(* Logix 5000 AddOnInstructionDefinition export; software revision 16.04 *)

TYPE ST_IOL_Error :   // IO-Link error codes
STRUCT
   nCommunicationError : DINT;   // Communication error
   nBlockError : INT;   // Function block error
   nIOLMError : INT;   // IO-Link master error
   nIOLError : INT;   // IO-Link device error
   iISDUIndex : DINT;   // IO-Link ISDU number
END_STRUCT
END_TYPE

TYPE STRING16 :   // string type
STRUCT
   LEN : DINT;
   DATA : SINT[16];
END_STRUCT
END_TYPE

TYPE STRING64 :   // string type
STRUCT
   LEN : DINT;
   DATA : SINT[64];
END_STRUCT
END_TYPE

TYPE STRING5 :   // string type
STRUCT
   LEN : DINT;
   DATA : SINT[5];
END_STRUCT
END_TYPE

TYPE ST_IOL_Data :   // Message elements and IO-Link record
STRUCT
   msgSource : SINT[255];   // Message: Source element
   msgDestination : SINT[255];   // Message: Destination element
   IOL_Record : SINT[232];   // IO-Link Record
END_STRUCT
END_TYPE

TYPE STRING8 :   // string type
STRUCT
   LEN : DINT;
   DATA : SINT[8];
END_STRUCT
END_TYPE

TYPE ST_PARKER_P8S :   // This data type includes the values of the IO-Link device
STRUCT
   VendorName : STRING16;   // ISDU 16: Vendor Name [String]
   ProductName : STRING16;   // ISDU 18: Product Name [String]
   VendorText : STRING64;   // ISDU 17: Vendor Text [String]
   ProductID : STRING64;   // ISDU 19: Product ID [String]
   ProductText : STRING64;   // ISDU 20: Product Text [String]
   SerialNumber : STRING8;   // ISDU 21: Serial Number [String]
   HWVersion : STRING5;   // ISDU 22: Hardware Version [String]
   FWVersion : STRING5;   // ISDU 23: Firmware Version [String]
   AppliName : STRING16;   // ISDU 24: Application Specific Tag [String]
   SysCommand : SINT;   // ISDU 2: Standard Command [Unsigned Integer]
   KeyLock : SINT;   // ISDU 81: Key Lock [Unsigned Integer]
END_STRUCT
END_TYPE

ADD_ON_INSTRUCTION FB_IOL_CALL_EIP   (* revision 3.1, vendor IO-Link *)
// This routine supports the communication between an IO-Link master and a Rockwell PLC via Ethernet/IP.
// Help:
// This routine supports the communication between an IO-Link master and a Rockwell PLC via Ethernet/IP. It makes it possible to read or write IO-Link variables (ISDUs) adressed via index and subindex.
// The function block supports the following EtherNet/IP IO-Link Masters:
// - SICK IOLG2EI (MasterType 0)
// - Balluff BNI EIP (MasterType 0)
// - Phoenix Axioline (MasterType 1)
// - Comtrol IOLM (MasterType 2)
// - Rockwell 1743-4IOL (MasterType 3)
VAR_IN_OUT
   msgCommunication_1 : MESSAGE; {required}   // Message instance for communication 1
   msgCommunication_2 : MESSAGE; {required}   // Message instance for communication 2
END_VAR
VAR_INPUT
   MasterType : SINT; {required}   // Type of the IO-Link master (0= SICK Master)
   PortNumber : SINT; {required}   // IO-Link port number (starting with 1)
   TimeOut : DINT; {visible}   // Time out time in [ms]
   Req : BOOL; {visible}   // Starts a request by a rising edge
   RW : BOOL; {visible}   // Read/Write selection (0= Read/ 1=Write)
   IOLIndex : DINT; {visible}   // IO-Link Index
   IOLSubIndex : INT; {visible}   // IO-Link Sub-Index
   Length : DINT; {visible}   // Byte-Length of the data that shold be written
END_VAR
VAR_OUTPUT
   ReadLength : DINT; {visible}   // Byte-Length of the read data
   Done : BOOL; {visible}   // Job done
   Busy : BOOL; {visible}   // Job busy
   Error : BOOL; {visible}   // Error detected (see Errorcode for more details)
END_VAR
VAR_IN_OUT
   Errorcode : ST_IOL_Error; {required}
   Data : ST_IOL_Data; {required}   // Data
END_VAR
VAR
   stTempError : ST_IOL_Error;
   iTemp1 : INT;   // Temporariliy variable
   iStep : INT;   // Current AOI step
   fbTriggerReq : FBD_ONESHOT;   // Instance: Edge detection (Req)
   fbTriggerMsgError2 : FBD_ONESHOT;   // Instance: Edge detection (MsgError2)
   fbTriggerMsgError1 : FBD_ONESHOT;   // Instance: Edge detection (MsgError1)
   fbTimeOut : FBD_TIMER;   // Instance: Time out
END_VAR

ROUTINE Logic   (* structured text *)
   (*=================================================================================
   Name: FB_IOL_Call_EIP
   Author: IO-Link
   -----------------------------------------------------------------------------------
   Description:
   This AOI supports the communication between an IO-Link master and a Rockwell
   PLC via Ethernet/IP. It makes it possible to read or write IO-Link variables (ISDUs)
   addressed via index and subindex.
   
   The function block supports the following EtherNet/IP IO-Link Masters:
   - SICK IOLG2EI          (MasterType 0)
   - Balluff BNI EIP       (MasterType 0)
   - Phoenix Axioline      (MasterType 1)
   - Comtrol IOLM          (MasterType 2)
   - Rockwell 1743-4IOL    (MasterType 3)
   
   -----------------------------------------------------------------------------------
   Version history:
   Date        | Version | Author  | Remark
   -----------------------------------------------------------------------------------
   03/08/2015  | 1.0     | IO-Link | Release version
   12/10/2015  | 2.0     | IO-Link | Support Phoenix IOLM
   04/02/2016  | 2.1     | IO-Link | Support Comtrol IOLM
   01/04/2016  | 2.2     | IO-Link | Support RA 1734 4IOL
   30/11/2016  | 3.0     | IO-Link | Error code extension
   25/04/2017  | 3.1     | IO-Link | Fix blocking of the MSG boxes
   ==================================================================================*)
   
   
   (*========== General ==========*)
   (*Initialize*)
   IF s:Fs THEN
   	Done:= 0;
   	Busy:= 0;
   	Error:= 0;
   	Errorcode.nCommunicationError:= 0;
   	Errorcode.nBlockError:= 0;
   	Errorcode.nIOLMError:= 0;
   	Errorcode.nIOLError:= 0;
   	Errorcode.iISDUIndex:= 0;
   	iStep:= 0;
   END_IF;
   
   (*Rising edge detection*)
   fbTriggerReq.InputBit:= Req;
   fbTriggerMsgError1.InputBit:= msgCommunication_1.ER;
   fbTriggerMsgError2.InputBit:= msgCommunication_2.ER;
   OSRI(fbTriggerReq);
   OSRI(fbTriggerMsgError1);
   OSRI(fbTriggerMsgError2);
   
   (*Error detetion*)
   IF (stTempError.nCommunicationError <>0 OR stTempError.nBlockError <>0 OR stTempError.nIOLMError <>0 OR stTempError.nIOLError <>0) AND Busy THEN
   	Errorcode.nCommunicationError:= stTempError.nCommunicationError;
   	Errorcode.nBlockError:= stTempError.nBlockError;
   	Errorcode.nIOLMError:= stTempError.nIOLMError;
   	Errorcode.nIOLError:= stTempError.nIOLError;
   	Errorcode.iISDUIndex:= stTempError.iISDUIndex;
   	stTempError.nCommunicationError:= 0;
   	stTempError.nBlockError:= 0;
   	stTempError.nIOLMError:= 0;
   	stTempError.nIOLError:= 0;
   	stTempError.iISDUIndex:= 0;
   
   	Done:= 0;
   	Busy:= 0;
   	Error:= 1;
   	iStep:= 0;
   	TND();
   END_IF;
   
   (*Time out detection*)
   fbTimeOut.TimerEnable:= Busy;
   fbTimeOut.PRE:= TimeOut;
   TONR(fbTimeOut);
   IF fbTimeOut.DN THEN
   	stTempError.nBlockError:= 16#0900; (*Error: Timeout*)
   	stTempError.iISDUIndex:= IOLIndex;
   	TND();
   END_IF;
   
   (*Get explicit messaging errors*)
   IF fbTriggerMsgError1.OutputBit THEN
   	stTempError.nCommunicationError:= (msgCommunication_1.EXERR * 65536) XOR msgCommunication_1.ERR;
   	stTempError.iISDUIndex:= IOLIndex;
   	TND();
   END_IF;
   
   (*Get explicit messaging errors*)
   IF fbTriggerMsgError2.OutputBit THEN
   	stTempError.nCommunicationError:= (msgCommunication_2.EXERR * 65536) XOR msgCommunication_2.ERR;
   	stTempError.iISDUIndex:= IOLIndex;
   	TND();
   END_IF;
   
   (*========== Send a new request ==========*)
   IF fbTriggerReq.OutputBit AND NOT Busy THEN
   	Done:= 0;
   	Busy:= 1;
   	Error:= 0;
   	Errorcode.nCommunicationError:= 0;
   	Errorcode.nBlockError:= 0;
   	Errorcode.nIOLMError:= 0;
   	Errorcode.nIOLError:= 0;
   	Errorcode.iISDUIndex:= 0;
   
   	iStep:= 1; (*Next step*)
   	TND();
   END_IF;
   
   
   (*========== Check parameter values ==========*)
   IF iStep =1 THEN
   
   	(*Check time out time*)
   	IF TimeOut <= 0 THEN
   		stTempError.nBlockError:= 16#0800; (*Error: Invalid time out time*)
   		stTempError.iISDUIndex:= IOLIndex;
   		TND();
   
   	(*Check port number*)
   	ELSIF PortNumber < 1 THEN
   		stTempError.nBlockError:= 16#0400; (*Error: Port number < 1*)
   		stTempError.iISDUIndex:= IOLIndex;
   		TND();
   
   	(*Check index*)
   	ELSIF IOLIndex < 0 OR IOLIndex > 32767 THEN
   		stTempError.nBlockError:= 16#0100; (*Error: 0 > Index > 32767*)
   		stTempError.iISDUIndex:= IOLIndex;
   		TND();
   
   	(*Check sub-index*)
   	ELSIF IOLSubIndex < 0 OR IOLSubIndex >255 THEN
   		stTempError.nBlockError:= 16#0300; (*Error: 0 > Sub-Index > 255*)
   		stTempError.iISDUIndex:= IOLIndex;
   		TND();
   
   	(*Check length*)
   	ELSIF Length < 0 OR Length > 232 THEN
   		stTempError.nBlockError:= 16#0200; (*Error: 0 > Length > 232*)
   		stTempError.iISDUIndex:= IOLIndex;
   		TND();
   	END_IF;
   
   	(*Check master type*)
   	IF MasterType = 0 THEN (*SICK*)
   		iStep:= 10; (*Next step*)
   	ELSIF MasterType = 1 THEN (*Phoenix*)
   		iStep:= 20;
   	ELSIF MasterType = 2 THEN (*Comtrol*)
   		iStep:= 30;
   	ELSIF MasterType = 3 THEN (*RA*)
   		iStep:= 40;
   	ELSE
   		stTempError.nBlockError:= 16#0600; (*Error: Master type <> 0*)
   		TND();
   	END_IF;
   END_IF;
   
   
   (*********** SICK IO-Link Master***********)
   (*========== Send a request ==========*)
   IF iStep =10 AND NOT msgCommunication_1.EW AND NOT msgCommunication_1.ST THEN
   	(*Define message parameter*)
   	msgCommunication_1.Class:= 150; (*Fix 0x96*)
   	msgCommunication_1.Instance:= PortNumber; (*Port starts at 1*)
   
   	(*Define index and subindex*)
   	COP(IOLIndex, Data.msgSource[0], 2); (*Index*)
   	Data.msgSource[2]:= IOLSubIndex; (*Sub-Index*)
   
   	(*Add attribute and payload*)
   	IF RW THEN
   		msgCommunication_1.Attribute:= 2; (*Write ISDU*)
   		msgCommunication_1.REQ_LEN:= 3 + Length; (*Byte length of the request*)
   		COP(Data.IOL_Record[0], Data.msgSource[3],Length); (*Payload*)
   	ELSE
   		msgCommunication_1.Attribute:= 3; (*Read ISDU*)
   		msgCommunication_1.REQ_LEN:= 3; (*Byte length of the request*)
   	END_IF;
   
   	(*Send request*)
   	MSG(msgCommunication_1);
   	iStep:= 11; (*Next step*)
   	TND();
   END_IF;
   
   
   (*========== Wait for reponse ==========*)
   IF iStep =11 THEN
   	IF fbTriggerMsgError1.OutputBit THEN
   		stTempError.nCommunicationError:= (msgCommunication_1.EXERR * 65536) XOR msgCommunication_1.ERR;
   		TND();
   	ELSIF msgCommunication_1.DN THEN
   		(*Valid response*)
   		IF Data.msgDestination[0] = 0 THEN
   			(*Write response*)
   			IF msgCommunication_1.Attribute = 2 THEN
   				iStep:= 2; (*Next step*)
   
   			(*Read response*)
   			ELSIF msgCommunication_1.Attribute = 3 THEN
   				ReadLength:= msgCommunication_1.DN_LEN - 1; (*Length of the response data*)
   				COP(Data.msgDestination[1], Data.IOL_Record[0], ReadLength);
   				iStep:= 2; (*Next step*)
   			END_IF;
   
   		(*IO-Link error detected*)
   		ELSIF Data.msgDestination[0] = -128 THEN
   			COP(Data.msgDestination[1], iTemp1, 2); (*Error: IO-Link Master*)
   			SWPB(iTemp1, REVERSE,stTempError.nIOLMError);
   			COP(Data.msgDestination[3], iTemp1, 2); (*Error: IO-Link Device*)
   			SWPB(iTemp1, REVERSE,stTempError.nIOLError);
   			TND();
   
   		(*Invalid response*)
   		ELSE
   			stTempError.nBlockError:= 16#0500; (*Error: Unknown response*)
   			stTempError.iISDUIndex:= IOLIndex;
   			TND();
   		END_IF;
   	END_IF;
   END_iF;
   
   
   (*********** Phoenix IO-Link Master***********)
   (*========== Read/Write handling ==========*)
   IF iStep = 20 AND NOT msgCommunication_1.EW AND NOT msgCommunication_1.ST AND NOT msgCommunication_2.EW AND NOT msgCommunication_2.ST THEN
   	(*Define message parameter*)
   	msgCommunication_1.Class:= 128; (*Fix 0x80*)
   	msgCommunication_1.Instance:= 1; (*Fix*)
   	msgCommunication_1.Attribute:= PortNumber; (*Port starts at 1*)
   	msgCommunication_2.Class:= 128; (*Fix 0x80*)
   	msgCommunication_2.Instance:= 1; (*Fix*)
   	msgCommunication_2.Attribute:= PortNumber; (*Port starts at 1*)
   
   	(*Define index and subindex*)
   	COP(IOLIndex, Data.msgSource[0], 2); (*Index*)
   	Data.msgSource[2]:= IOLSubIndex; (*Sub-Index*)
   
   	IF RW THEN
   		iStep:= 23; (*Next step*)
   	ELSE
   		iStep:= 21; (*Next step*)
   	END_IF;
   END_IF;
   
   
   
   (*========== Read ISDU ==========*)
   IF iStep = 21 THEN
   	msgCommunication_1.REQ_LEN:= 3; (*Byte length of the request*)
   
   	(*Send request*)
   	MSG(msgCommunication_1);
   	iStep:= 22; (*Next step*)
   END_IF;
   
   
   (*========== Wait for read reponse ==========*)
   IF iStep = 22 THEN
   	IF fbTriggerMsgError1.OutputBit THEN
   		stTempError.nCommunicationError:= (msgCommunication_1.EXERR * 65536) XOR msgCommunication_1.ERR;
   		stTempError.iISDUIndex:= IOLIndex;
   		IF msgCommunication_1.ERR = 30 THEN
   			COP(Data.msgDestination[0], stTempError.nIOLMError, 2); (*Error: IO-Link Device*)
   			COP(Data.msgDestination[2], iTemp1, 2); (*Error: IO-Link Device*)
   			SWPB(iTemp1, REVERSE,stTempError.nIOLError);
   			TND();
   		END_IF;
   	ELSIF msgCommunication_1.DN THEN
   		ReadLength:= msgCommunication_1.DN_LEN; (*Length of the response data*)
   		COP(Data.msgDestination[0], Data.IOL_Record[0], ReadLength);
   		iStep:= 2; (*Next step*)
   	END_IF;
   END_IF;
   
   
   (*========== Write ISDU ==========*)
   IF iStep = 23 THEN
   	msgCommunication_2.REQ_LEN:= 3 + Length; (*Byte length of the request*)
   	COP(Data.IOL_Record[0], Data.msgSource[3],Length); (*Payload*)
   
   	(*Send request*)
   	MSG(msgCommunication_2);
   	iStep:= 24; (*Next step*)
   END_IF;
   
   
   (*========== Wait for write reponse ==========*)
   IF iStep = 24 THEN
   	IF fbTriggerMsgError2.OutputBit THEN
   		stTempError.nCommunicationError:= (msgCommunication_2.EXERR * 65536) XOR msgCommunication_2.ERR;
   		stTempError.iISDUIndex:= IOLIndex;
   		IF msgCommunication_2.ERR = 30 THEN
   			COP(Data.msgDestination[0], stTempError.nIOLMError, 2); (*Error: IO-Link Device*)
   			COP(Data.msgDestination[2], iTemp1, 2); (*Error: IO-Link Device*)
   			SWPB(iTemp1, REVERSE,stTempError.nIOLError);
   			TND();
   		END_IF;
   	ELSIF msgCommunication_2.DN THEN
   		iStep:= 2; (*Next step*)
   	END_IF;
   END_IF;
   
   
   (*********** Comtrol IO-Link Master***********)
   (*========== Send a request ==========*)
   IF iStep = 30 AND NOT msgCommunication_1.EW AND NOT msgCommunication_1.ST THEN
   	(*Define message parameter*)
   	msgCommunication_1.Class:= 116; (*Fix 0x74*)
   	msgCommunication_1.Instance:= PortNumber; (*Port starts at 1*)
   	msgCommunication_1.Attribute:= 1; (*Fix*)
   	Data.msgSource[0]:= 0; (*No byte swapping*)
   
   	(*Define index and subindex*)
   	COP(IOLIndex, Data.msgSource[2], 2); (*Index*)
   	Data.msgSource[4]:= IOLSubIndex; (*Sub-Index*)
   	Data.msgSource[5]:= 0; (*Sub-Index*)
   	msgCommunication_1.REQ_LEN:= 240; (*Byte length of the request = 232 + 8*)
   
   	(*Add attribute and payload*)
   	IF RW THEN
   		Data.msgSource[1]:= 2; (*Write operation*)
   		COP(Length, Data.msgSource[6], 2); (*Length*)
   		COP(Data.IOL_Record[0], Data.msgSource[8], Length); (*Payload*)
   	ELSE
   		Data.msgSource[1]:= 1; (*Read operation*)
   		Data.msgSource[6]:= -24; (*Max IO-Link length*)
   		Data.msgSource[7]:= 0;
   	END_IF;
   
   	(*Send request*)
   	MSG(msgCommunication_1);
   	iStep:= 31; (*Next step*)
   	TND();
   END_IF;
   
   
   (*========== Wait for reponse ==========*)
   IF iStep = 31 THEN
   	IF fbTriggerMsgError1.OutputBit THEN
   		stTempError.nCommunicationError:= (msgCommunication_1.EXERR * 65536) XOR msgCommunication_1.ERR;
   		stTempError.iISDUIndex:= IOLIndex;
   		TND();
   	ELSIF msgCommunication_1.DN THEN
   		(*Valid response*)
   		IF Data.msgDestination[0] = 32 THEN
   			(*Write response*)
   			IF Data.msgDestination[1] = 2 THEN
   				iStep:= 2; (*Next step*)
   
   			(*Read response*)
   			ELSIF Data.msgDestination[1] = 1 THEN
   				ReadLength:= Data.msgDestination[6];
   				COP(Data.msgDestination[8], Data.IOL_Record[0], ReadLength);
   				iStep:= 2; (*Next step*)
   			ELSE
   				stTempError.nBlockError:= 16#0500; (*Error: Unknown response*)
   				stTempError.iISDUIndex:= IOLIndex;
   				TND();
   			END_IF;
   
   		(*IOLM error detected*)
   		ELSIF Data.msgDestination[0] = 48 THEN
   			stTempError.nBlockError:= 16#000A; (*Error: Failure: IO-Link device rejected the request*)
   			stTempError.iISDUIndex:= IOLIndex;
   			TND();
   
   		ELSIF Data.msgDestination[0] = 64 THEN
   			stTempError.nBlockError:= 16#000B; (*Error: Timed out: IO-Link device did not respond*)
   			stTempError.iISDUIndex:= IOLIndex;
   			TND();
   
   		(*Invalid response*)
   		ELSE
   			stTempError.nBlockError:= 16#0500; (*Error: Unknown response*)
   			stTempError.iISDUIndex:= IOLIndex;
   			TND();
   		END_IF;
   	END_IF;
   END_iF;
   
   
   (*********** RA 1734 4IOL IO-Link Master***********)
   (*========== Read/Write handling ==========*)
   IF iStep = 40 AND NOT msgCommunication_1.EW AND NOT msgCommunication_1.ST AND NOT msgCommunication_2.EW AND NOT msgCommunication_2.ST THEN
   	(*Define message parameter*)
   	msgCommunication_1.Class:= 931; (*Fix 0x3A3*)
   	msgCommunication_1.Instance:= IOLIndex; (*I0-Link index*)
   	msgCommunication_1.Attribute:= 0; (*Fix*)
   	msgCommunication_2.Class:= 931; (*Fix 0x3A3*)
   	msgCommunication_2.Instance:= IOLIndex; (*I0-Link index*)
   	msgCommunication_2.Attribute:= 0; (*Fix*)
   
   	(*Define index and subindex*)
   	iTemp1:= PortNumber - 1;
   	Data.msgSource[0]:= IOLSubIndex; (*IO-Link subindex*)
   	Data.msgSource[1]:= PortNumber - 1; (*Port number*)
   
   	IF RW THEN
   		iStep:= 43; (*Next step*)
   	ELSE
   		iStep:= 41; (*Next step*)
   	END_IF;
   END_IF;
   
   
   (*========== Read ISDU ==========*)
   IF iStep = 41 THEN
   	msgCommunication_1.REQ_LEN:= 2; (*Byte length of the request*)
   
   	(*Send request*)
   	MSG(msgCommunication_1);
   	iStep:= 42; (*Next step*)
   END_IF;
   
   
   (*========== Wait for read reponse ==========*)
   IF iStep =42 THEN
   	IF fbTriggerMsgError1.OutputBit THEN
   		stTempError.nCommunicationError:= (msgCommunication_1.EXERR * 65536) XOR msgCommunication_1.ERR;
   		stTempError.iISDUIndex:= IOLIndex;
   		IF msgCommunication_1.ERR = 30 THEN
   			//COP(Data.msgDestination[0], stTempError.nIOLMError, 2); (*Error: IO-Link Device*)
   			//COP(Data.msgDestination[2], iTemp1, 2); (*Error: IO-Link Device*)
   			//SWPB(iTemp1, REVERSE, stTempError.nIOLError);
   			TND();
   		END_IF;
   	ELSIF msgCommunication_1.DN THEN
   		ReadLength:= msgCommunication_1.DN_LEN; (*Length of the response data*)
   		COP(Data.msgDestination[0], Data.IOL_Record[0], ReadLength);
   		iStep:= 2; (*Next step*)
   	END_IF;
   END_IF;
   
   
   (*========== Write ISDU ==========*)
   IF iStep = 43 THEN
   	msgCommunication_2.REQ_LEN:= 2 + Length; (*Byte length of the request*)
   	COP(Data.IOL_Record[0], Data.msgSource[2], Length); (*Payload*)
   
   	(*Send request*)
   	MSG(msgCommunication_2);
   	iStep:= 44; (*Next step*)
   END_IF;
   
   
   (*========== Wait for write reponse ==========*)
   IF iStep = 44 THEN
   	IF fbTriggerMsgError2.OutputBit THEN
   		stTempError.nCommunicationError:= (msgCommunication_2.EXERR * 65536) XOR msgCommunication_2.ERR;
   		stTempError.iISDUIndex:= IOLIndex;
   		IF msgCommunication_2.ERR =30 THEN
   			//COP(Data.msgDestination[0], stTempError.nIOLMError, 2); (*Error: IO-Link Device*)
   			//COP(Data.msgDestination[2], iTemp1, 2); (*Error: IO-Link Device*)
   			//SWPB(iTemp1, REVERSE, stTempError.nIOLError);
   			TND();
   		END_IF;
   	ELSIF msgCommunication_2.DN THEN
   		iStep:= 2; (*Next step*)
   	END_IF;
   END_IF;
   
   
   (*========== Job done ==========*)
   IF iStep =2 THEN
   	Done:= 1;
   	Busy:= 0;
   	Error:= 0;
   	Errorcode.nCommunicationError:= 0;
   	Errorcode.nBlockError:= 0;
   	Errorcode.nIOLMError:= 0;
   	Errorcode.nIOLError:= 0;
   	Errorcode.iISDUIndex:= 0;
   	iStep:= 0; (*Next step*)
   END_IF;
   
END_ROUTINE
END_ADD_ON_INSTRUCTION

ADD_ON_INSTRUCTION F_IOL_Internal17   (* revision 1.0, vendor IO-Link *)
// IO-Link internal AOI
// Revision note:
// Release version
// Help:
// IO-Link internal function. Please use this AOI only in combination with an IO-Link service data AOI.
VAR_INPUT
   bIsComplex : BOOL; {required}   // Data type is part of an complex data type e.g. record or array
END_VAR
VAR_IN_OUT
   arrTempItem : SINT[232]; {required}   // Temporariliy IO-Link Record
   arrIOLRecord : SINT[232]; {required}   // IO-Link Record
END_VAR
VAR_INPUT
   iFixedLength : INT; {required}
END_VAR
VAR_IN_OUT
   arrSourceData : SINT[1]; {required}
   iSourceLen : DINT; {required}
END_VAR
VAR
   iMaxStringLength : DINT;
   iIndex : DINT;
END_VAR

ROUTINE Logic   (* structured text *)
   (*Get max string length*)
   SIZE(arrSourceData[0], 0, iMaxStringLength);
   
   IF (iMaxStringLength >=iFixedLength) AND iFixedLength >0 AND iFixedLength <=232 THEN
   	(*Is part of an record or an array data type*)
   	IF bIsComplex THEN
   		FOR iIndex:= 0 TO iFixedLength-1 DO
   			IF iSourceLen < iFixedLength-iIndex THEN
   				arrTempItem[iIndex]:= 16#00;
   			ELSE
   				arrTempItem[iIndex]:= arrSourceData[iFixedLength-1-iIndex];
   			END_IF;
   		END_FOR;
   
   	(*Is a simple data type*)
   	ELSE
   		FOR iIndex:= 0 TO iFixedLength-1 DO
   			IF iIndex <= iSourceLen-1 THEN
   				arrIOLRecord[iIndex]:= arrSourceData[iIndex];
   			ELSE
   				arrIOLRecord[iIndex]:= 16#00;
   			END_IF;
   		END_FOR;
   	END_IF;
   END_IF;
END_ROUTINE
END_ADD_ON_INSTRUCTION

ADD_ON_INSTRUCTION F_IOL_Internal8   (* revision 1.0, vendor IO-Link *)
// IO-Link internal AOI
// Revision note:
// Release version
// Help:
// IO-Link internal function. Please use this AOI only in combination with an IO-Link service data AOI.
VAR_INPUT
   bIsComplex : BOOL; {required}   // Data type is part of an complex data type e.g. record or array
END_VAR
VAR_IN_OUT
   arrTempItem : SINT[232]; {required}   // Temporariliy IO-Link Record
   arrIOLRecord : SINT[232]; {required}   // IO-Link Record
END_VAR
VAR_INPUT
   iFixedLength : INT; {required}
END_VAR
VAR_IN_OUT
   arrDestinationData : SINT[1]; {required}
   iDestinationLen : DINT; {required}
END_VAR
VAR
   iStringLength : DINT;
   iIndex : DINT;
END_VAR

ROUTINE Logic   (* structured text *)
   (*Inititalization*)
   iStringLength:= 0;
   
   (*Calculate the actual string length*)
   IF iFixedLength <= 232 THEN
   	FOR iIndex:=0 TO iFixedLength-1 DO
   		IF bIsComplex THEN
   			IF arrTempItem[iIndex] = 16#0 THEN
   				EXIT;
   			ELSE
   				iStringLength:= iStringLength + 1;
   			END_IF;
   		ELSE
   			IF arrIOLRecord[iIndex] = 16#0 THEN
   				EXIT;
   			ELSE
   				iStringLength:= iStringLength + 1;
   			END_IF;
   		END_IF;
   	END_FOR;
   
   	(*Copy to the return value*)
   	IF bIsComplex THEN
   		COP(arrTempItem[0], arrDestinationData[0], iStringLength);
   	ELSE
   		COP(arrIOLRecord[0], arrDestinationData[0], iStringLength);
   	END_IF;
   
   	(*Add string length*)
   	iDestinationLen:= iStringLength;
   ELSE
     iDestinationLen:= 0;
   END_IF;
END_ROUTINE
END_ADD_ON_INSTRUCTION

ADD_ON_INSTRUCTION FB_PARKER_P8S_EIP   (* revision 1.6, vendor Parker Hannifin GmbH *)
// PARKER FB_PARKER_P8S service data IO-Link AOI
// Revision note:
// Generator version: 1.9.0.1000R
// Help:
// The main goal of the Add-On Instruction is to facilitate establishing acyclic communication with PARKER IO-Link devices. It shell not be necessary for the most important devices parameters to know their indices. The AOI can be used several times in the project. This AOI is only suitable with RSLogix5000 V16 or higher. The device's most important parameters will be offered as inputs.
VAR_IN_OUT
   msgCommunication_1 : MESSAGE; {required}   // Communication message instance 1
   msgCommunication_2 : MESSAGE; {required}   // Communication message instance 2
   stIolCallData : ST_IOL_Data; {required}   // IO-Link call data
END_VAR
VAR_INPUT
   MasterType : SINT; {visible}   // Type of the IO-Link master (0= SICK/Balluff IOLM, 1=Phoenix IOLM, 2=Comtrol IOLM)
   PortNumber : SINT; {visible}   // IO-Link port number (starting with 1)
   TimeOut : DINT; {visible}   // Time out time in [ms]
   Req : BOOL; {visible}   // Positive edge: Carry out data transfer
   RW : BOOL; {visible}   // Read or write operation (FALSE=Read, TRUE=Write)
   VendorName : BOOL; {visible}   // Vendor Name (ISDU:16) RO-Access
   ProductName : BOOL; {visible}   // Product Name (ISDU:18) RO-Access
   VendorText : BOOL; {visible}   // Vendor Text (ISDU:17) RO-Access
   ProductID : BOOL; {visible}   // Product ID (ISDU:19) RO-Access
   ProductText : BOOL; {visible}   // Product Text (ISDU:20) RO-Access
   SerialNumber : BOOL; {visible}   // Serial Number (ISDU:21) RO-Access
   HWVersion : BOOL; {visible}   // Hardware Version (ISDU:22) RO-Access
   FWVersion : BOOL; {visible}   // Firmware Version (ISDU:23) RO-Access
   AppliName : BOOL; {visible}   // Application Specific Tag (ISDU:24) RW-Access
   SysCommand : BOOL; {visible}   // Standard Command (ISDU:2) WO-Access
   KeyLock : BOOL; {visible}   // Key Lock (ISDU:81) RW-Access
END_VAR
VAR_IN_OUT
   DeviceData : ST_PARKER_P8S; {required}   // Reference to the device data tag
END_VAR
VAR_OUTPUT
   Done : BOOL; {visible}   // Job done
   Busy : BOOL; {visible}   // Request in process
   Error : BOOL; {visible}   // Error occured
END_VAR
VAR_IN_OUT
   Errorcode : ST_IOL_Error; {required}   // Error code
END_VAR
VAR
   fbIolCall : FB_IOL_CALL_EIP;   // IO-Link call reference
   fbTriggerDone : FBD_ONESHOT;   // Rising edge detection
   fbTriggerError : FBD_ONESHOT;   // Rising edge detection
   fbTriggerReq : FBD_ONESHOT;   // Rising edge detection
   fbTimeOut : FBD_TIMER;   // Time out detection
   stIolCallError : ST_IOL_Error;   // IO-Link call error
   stLastErrorCode : ST_IOL_Error;   // Last error code
   bRWSave : BOOL;   // Backup of the Read/Write flag
   iNumSelection : INT;   // Number of selected input options
   iStep : INT;   // Current AOI step
   iCommandIndex : INT;   // Current command index
   iIndex : INT;   // Temporarily index variable
   iTemp : INT;   // Temporarily variable
   arrInputSelection : BOOL[32];   // Backup of the input options
   arrTempItem : SINT[232];   // Temporarily data
   arrTemp : SINT[4];   // Temporarily variable
   BlockIdentifier : DINT;   // Block identifier
   arrCommandQueue : INT[15];   // Command queue
   fbInternal8 : F_IOL_Internal8;   // Instance of the internal IO-Link function
   fbInternal17 : F_IOL_Internal17;   // Instance of the internal IO-Link function
END_VAR

ROUTINE Logic   (* structured text *)
   (*=================================================================================
   Name: P8S IO-Link service data Add-On Instruction
   Company: Parker Hannifin GmbH
   Date: Wed Apr 25 10:59:19 CEST 2018
   Generator Version: V1.9.0.1000R
   IODD Version: V1.3
   -----------------------------------------------------------------------------------
   Description:
   The main goal of the Add-On Instruction is to facilitate establishing acyclic
   communication with PARKER IO-Link devices. It shell not be
   necessary for the most important devices parameters to know their indices. The AOI
   can be used several times in the project. This AOI is only suitable with
   RSLogix5000 V16 or higher. The device's most important parameters will be offered
   as inputs.
   =================================================================================*)
   
   (*Communication*)
   FB_IOL_CALL_EIP(fbIolCall, msgCommunication_1, msgCommunication_2, MasterType, PortNumber, stIolCallError, stIolCallData);
   fbIolCall.Req:= 0;
   
   (*Create rising edge flags*)
   fbTriggerDone.InputBit:= fbIolCall.Done;
   fbTriggerError.InputBit:= fbIolCall.Error;
   fbTriggerReq.InputBit:= Req;
   OSRI(fbTriggerDone);
   OSRI(fbTriggerError);
   OSRI(fbTriggerReq);
   
   (*Block identifier*)
   BlockIdentifier:= 491;
   
   (*Create IEC timer*)
   fbTimeOut.TimerEnable:= Busy;
   fbTimeOut.PRE:= TimeOut;
   TONR(fbTimeOut);
   
   (*Error management*)
   IF stLastErrorCode.nBlockError <> 16#0 OR stLastErrorCode.nCommunicationError <> 16#0 OR stLastErrorCode.nIOLMError <> 16#0 OR stLastErrorCode.nIOLError <> 16#0 THEN
   	Done:= 0;
   	Busy:= 0;
   	Error:= 1;
   	Errorcode.nCommunicationError:= stLastErrorCode.nCommunicationError;
   	Errorcode.nBlockError:= stLastErrorCode.nBlockError;
   	Errorcode.nIOLMError:= stLastErrorCode.nIOLMError;
   	Errorcode.nIOLError:= stLastErrorCode.nIOLError;
   	Errorcode.iISDUIndex:= stLastErrorCode.iISDUIndex;
   
   	stLastErrorCode.nCommunicationError:= 16#0000_0000;
   	stLastErrorCode.nBlockError:= 16#0000;
   	stLastErrorCode.nIOLMError:= 16#0000;
   	stLastErrorCode.nIOLError:= 16#0000;
   	stLastErrorCode.iISDUIndex:= 0;
   	iStep:= 0;
   	TND();
   END_IF;
   
   (*IOL-Call error detected*)
   IF fbTriggerError.OutputBit THEN
   	stLastErrorCode.nCommunicationError:= stIolCallError.nCommunicationError;
   	stLastErrorCode.nBlockError:= stIolCallError.nBlockError;
   	stLastErrorCode.nIOLMError:= stIolCallError.nIOLMError;
   	stLastErrorCode.nIOLError:= stIolCallError.nIOLError;
   	stLastErrorCode.iISDUIndex:= stIolCallError.iISDUIndex;
   	TND();
   END_IF;
   
   (*Time out detected*)
   IF fbTimeOut.DN THEN
   	stLastErrorCode.nBlockError:= 16#0009; // Error: Time out detected
   	TND();
   END_IF;
   
   
   
   (*Create command queue*)
   IF fbTriggerReq.OutputBit AND NOT Busy THEN
   	// Status update
   	Done:= 0;
   	Busy:= 1;
   	Error:= 0;
   	Errorcode.nCommunicationError:= 16#0000_0000;
   	Errorcode.nBlockError:= 16#0000;
   	Errorcode.nIOLMError:= 16#0000;
   	Errorcode.nIOLError:= 16#0000;
   	Errorcode.iISDUIndex:= 0;
   	stLastErrorCode.nCommunicationError:= 16#0000_0000;
   	stLastErrorCode.nBlockError:= 16#0000;
   	stLastErrorCode.nIOLMError:= 16#0000;
   	stLastErrorCode.nIOLError:= 16#0000;
   	stLastErrorCode.iISDUIndex:= 0;
   
   	bRWSave:= RW;
   	iCommandIndex:= 0;
   
   	// Initialize command queue
   	FOR iIndex:= 0 TO 14 DO
   		arrCommandQueue[iIndex]:= -1;
   	END_FOR;
   
   	// Check number of parameter selection
   	iNumSelection:= 0;
   
   	arrInputSelection[0]:= VendorName;
   	arrInputSelection[1]:= ProductName;
   	arrInputSelection[2]:= VendorText;
   	arrInputSelection[3]:= ProductID;
   	arrInputSelection[4]:= ProductText;
   	arrInputSelection[5]:= SerialNumber;
   	arrInputSelection[6]:= HWVersion;
   	arrInputSelection[7]:= FWVersion;
   	arrInputSelection[8]:= AppliName;
   	arrInputSelection[9]:= SysCommand;
   	arrInputSelection[10]:= KeyLock;
   
   	FOR iIndex:= 0 TO 10 DO
   		IF arrInputSelection[iIndex] THEN
   			iNumSelection:= iNumSelection + 1;
   		END_IF;
   	END_FOR;
   
   	(*Create command queue*)
   	iIndex:= 0;
   
   	IF VendorName THEN
   		IF  bRWSave THEN
   			stLastErrorCode.nBlockError:= 16#0004; // Error: Parameter is not writable
   			stLastErrorCode.iISDUIndex:= 16;
   		ELSE
   			arrCommandQueue[iIndex]:= 16;
   			iIndex:= iIndex + 1;
   		END_IF;
   	END_IF;
   
   	IF ProductName THEN
   		IF  bRWSave THEN
   			stLastErrorCode.nBlockError:= 16#0004; // Error: Parameter is not writable
   			stLastErrorCode.iISDUIndex:= 18;
   		ELSE
   			arrCommandQueue[iIndex]:= 18;
   			iIndex:= iIndex + 1;
   		END_IF;
   	END_IF;
   
   	IF VendorText THEN
   		IF  bRWSave THEN
   			stLastErrorCode.nBlockError:= 16#0004; // Error: Parameter is not writable
   			stLastErrorCode.iISDUIndex:= 17;
   		ELSE
   			arrCommandQueue[iIndex]:= 17;
   			iIndex:= iIndex + 1;
   		END_IF;
   	END_IF;
   
   	IF ProductID THEN
   		IF  bRWSave THEN
   			stLastErrorCode.nBlockError:= 16#0004; // Error: Parameter is not writable
   			stLastErrorCode.iISDUIndex:= 19;
   		ELSE
   			arrCommandQueue[iIndex]:= 19;
   			iIndex:= iIndex + 1;
   		END_IF;
   	END_IF;
   
   	IF ProductText THEN
   		IF  bRWSave THEN
   			stLastErrorCode.nBlockError:= 16#0004; // Error: Parameter is not writable
   			stLastErrorCode.iISDUIndex:= 20;
   		ELSE
   			arrCommandQueue[iIndex]:= 20;
   			iIndex:= iIndex + 1;
   		END_IF;
   	END_IF;
   
   	IF SerialNumber THEN
   		IF  bRWSave THEN
   			stLastErrorCode.nBlockError:= 16#0004; // Error: Parameter is not writable
   			stLastErrorCode.iISDUIndex:= 21;
   		ELSE
   			arrCommandQueue[iIndex]:= 21;
   			iIndex:= iIndex + 1;
   		END_IF;
   	END_IF;
   
   	IF HWVersion THEN
   		IF  bRWSave THEN
   			stLastErrorCode.nBlockError:= 16#0004; // Error: Parameter is not writable
   			stLastErrorCode.iISDUIndex:= 22;
   		ELSE
   			arrCommandQueue[iIndex]:= 22;
   			iIndex:= iIndex + 1;
   		END_IF;
   	END_IF;
   
   	IF FWVersion THEN
   		IF  bRWSave THEN
   			stLastErrorCode.nBlockError:= 16#0004; // Error: Parameter is not writable
   			stLastErrorCode.iISDUIndex:= 23;
   		ELSE
   			arrCommandQueue[iIndex]:= 23;
   			iIndex:= iIndex + 1;
   		END_IF;
   	END_IF;
   
   	IF AppliName THEN
   		arrCommandQueue[iIndex]:= 24;
   		iIndex:= iIndex + 1;
   	END_IF;
   
   	IF SysCommand THEN
   		IF NOT bRWSave THEN
   			stLastErrorCode.nBlockError:= 16#0003; // Error: Parameter is not readable
   			stLastErrorCode.iISDUIndex:= 2;
   		ELSE
   			arrCommandQueue[iIndex]:= 2;
   			iIndex:= iIndex + 1;
   		END_IF;
   	END_IF;
   
   	IF KeyLock THEN
   		arrCommandQueue[iIndex]:= 81;
   		iIndex:= iIndex + 1;
   	END_IF;
   
   
   	// Next step
   	IF stLastErrorCode.nBlockError = 0 THEN
   		iStep:= 1;
   	END_IF;
   	TND(); // Show the Busy-Flag for minimum one PLC cycle
   END_IF;
   
   (*Check input selection*)
   IF iStep = 1 THEN
   	IF iNumSelection = 0 THEN
   		stLastErrorCode.nBlockError:= 16#0002;  // Error: No parameter selected
   		TND();
   	END_IF;
   
   	// Next step
   	iStep:= 2;
   END_IF;
   
   (*Send telegram to the IO-Link device*)
   IF iStep = 2 AND NOT fbIolCall.BUSY AND Busy THEN
   	CASE arrCommandQueue[iCommandIndex] OF
   	(*(16) Vendor Name*)
   	16:
   	fbIolCall.Length:= 16;
   	fbIolCall.RW:= bRWSave;
   	fbIolCall.IOLIndex:= 16;
   
   	(*(18) Product Name*)
   	18:
   	fbIolCall.Length:= 16;
   	fbIolCall.RW:= bRWSave;
   	fbIolCall.IOLIndex:= 18;
   
   	(*(17) Vendor Text*)
   	17:
   	fbIolCall.Length:= 64;
   	fbIolCall.RW:= bRWSave;
   	fbIolCall.IOLIndex:= 17;
   
   	(*(19) Product ID*)
   	19:
   	fbIolCall.Length:= 64;
   	fbIolCall.RW:= bRWSave;
   	fbIolCall.IOLIndex:= 19;
   
   	(*(20) Product Text*)
   	20:
   	fbIolCall.Length:= 64;
   	fbIolCall.RW:= bRWSave;
   	fbIolCall.IOLIndex:= 20;
   
   	(*(21) Serial Number*)
   	21:
   	fbIolCall.Length:= 8;
   	fbIolCall.RW:= bRWSave;
   	fbIolCall.IOLIndex:= 21;
   
   	(*(22) Hardware Version*)
   	22:
   	fbIolCall.Length:= 5;
   	fbIolCall.RW:= bRWSave;
   	fbIolCall.IOLIndex:= 22;
   
   	(*(23) Firmware Version*)
   	23:
   	fbIolCall.Length:= 5;
   	fbIolCall.RW:= bRWSave;
   	fbIolCall.IOLIndex:= 23;
   
   	(*(24) Application Specific Tag*)
   	24:
   	fbIolCall.Length:= 16;
   	fbIolCall.RW:= bRWSave;
   	fbIolCall.IOLIndex:= 24;
   
   	IF bRWSave THEN
   		F_IOL_Internal17(fbInternal17, 0, arrTempItem, stIolCallData.IOL_Record, 16, DeviceData.AppliName.DATA, DeviceData.AppliName.LEN);
   	END_IF;
   
   	(*(2) Standard Command*)
   	2:
   	fbIolCall.Length:= 1;
   	fbIolCall.RW:= bRWSave;
   	fbIolCall.IOLIndex:= 2;
   
   	IF bRWSave THEN
   		stIolCallData.IOL_Record[0]:= DeviceData.SysCommand;
   	END_IF;
   
   	(*(81) Key Lock*)
   	81:
   	fbIolCall.Length:= 1;
   	fbIolCall.RW:= bRWSave;
   	fbIolCall.IOLIndex:= 81;
   
   	IF bRWSave THEN
   		stIolCallData.IOL_Record[0]:= DeviceData.KeyLock;
   	END_IF;
   
   	END_CASE;
   
   	// Start IOL-Call FB
   	fbIolCall.Req:= 1;
   
   	// Next step
   	iStep:= 3;
   END_IF;
   
   (*Receive telegram from the IO-Link device*)
   IF iStep = 3 AND fbTriggerDone.OutputBit AND Busy THEN
   	IF NOT bRWSave THEN
   		CASE fbIolCall.IOLIndex OF
   		(*(16) Vendor Name*)
   		16:
   		F_IOL_Internal8(fbInternal8, 0, arrTempItem, stIolCallData.IOL_Record, fbIolCall.ReadLength, DeviceData.VendorName.DATA, DeviceData.VendorName.LEN);
   
   		(*(18) Product Name*)
   		18:
   		F_IOL_Internal8(fbInternal8, 0, arrTempItem, stIolCallData.IOL_Record, fbIolCall.ReadLength, DeviceData.ProductName.DATA, DeviceData.ProductName.LEN);
   
   		(*(17) Vendor Text*)
   		17:
   		F_IOL_Internal8(fbInternal8, 0, arrTempItem, stIolCallData.IOL_Record, fbIolCall.ReadLength, DeviceData.VendorText.DATA, DeviceData.VendorText.LEN);
   
   		(*(19) Product ID*)
   		19:
   		F_IOL_Internal8(fbInternal8, 0, arrTempItem, stIolCallData.IOL_Record, fbIolCall.ReadLength, DeviceData.ProductID.DATA, DeviceData.ProductID.LEN);
   
   		(*(20) Product Text*)
   		20:
   		F_IOL_Internal8(fbInternal8, 0, arrTempItem, stIolCallData.IOL_Record, fbIolCall.ReadLength, DeviceData.ProductText.DATA, DeviceData.ProductText.LEN);
   
   		(*(21) Serial Number*)
   		21:
   		F_IOL_Internal8(fbInternal8, 0, arrTempItem, stIolCallData.IOL_Record, fbIolCall.ReadLength, DeviceData.SerialNumber.DATA, DeviceData.SerialNumber.LEN);
   
   		(*(22) Hardware Version*)
   		22:
   		F_IOL_Internal8(fbInternal8, 0, arrTempItem, stIolCallData.IOL_Record, fbIolCall.ReadLength, DeviceData.HWVersion.DATA, DeviceData.HWVersion.LEN);
   
   		(*(23) Firmware Version*)
   		23:
   		F_IOL_Internal8(fbInternal8, 0, arrTempItem, stIolCallData.IOL_Record, fbIolCall.ReadLength, DeviceData.FWVersion.DATA, DeviceData.FWVersion.LEN);
   
   		(*(24) Application Specific Tag*)
   		24:
   		F_IOL_Internal8(fbInternal8, 0, arrTempItem, stIolCallData.IOL_Record, fbIolCall.ReadLength, DeviceData.AppliName.DATA, DeviceData.AppliName.LEN);
   
   
   		(*(81) Key Lock*)
   		81:
   		DeviceData.KeyLock:= stIolCallData.IOL_Record[0];
   
   		END_CASE;
   	END_IF;
   
   	// Select next command
   	iCommandIndex:= iCommandIndex + 1;
   
   	// Job done
   	IF (iCommandIndex > 14) OR (arrCommandQueue[iCommandIndex] = -1) THEN
   		Done:= 1;
   		Busy:= 0;
   		Error:= 0;
   		Errorcode.nCommunicationError:= 16#0000_0000;
   		Errorcode.nBlockError:= 16#0000;
   		Errorcode.nIOLMError:= 16#0000;
   		Errorcode.nIOLError:= 16#0000;
   		Errorcode.iISDUIndex:= 0;
   		iStep:= 0;
   
   	// Next command
   	ELSE
   		iStep:= 2; // Send next IO-Link request
   	END_IF;
   END_IF;
END_ROUTINE
END_ADD_ON_INSTRUCTION
